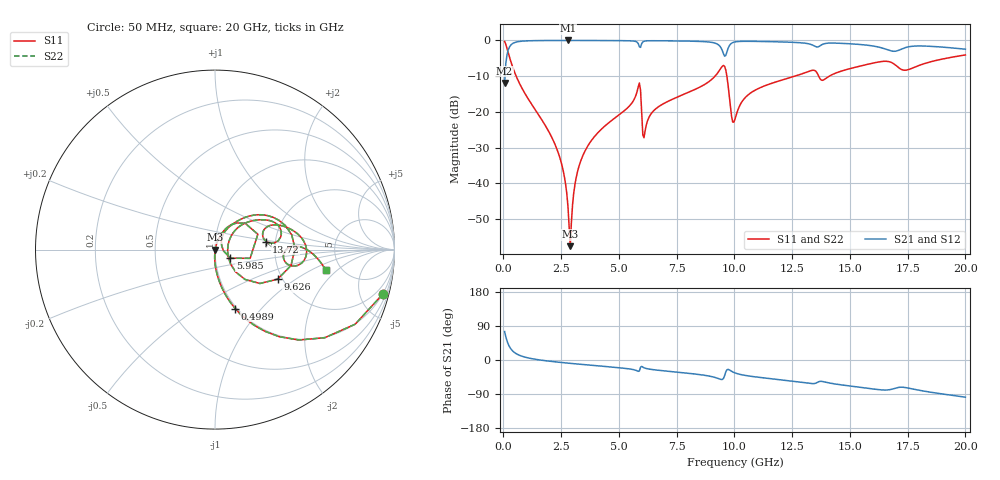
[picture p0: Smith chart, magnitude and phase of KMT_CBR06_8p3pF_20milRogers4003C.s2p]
! Data measured by Modelithics Inc. support@modelithics.com 813-866-6335
! KEMET CBR0603 8.3pF, Pad Width= 0.851mm, Pad Length= 0.64mm, Pad Gap= 0.62mm, 20mil Rogers 4003C substrate Data, January 2022
# hz S ma R 50
! 2 Port Network Data from SP1.SP block
! freq  magS11  angS11  magS21  angS21  magS12  angS12  magS22  angS22
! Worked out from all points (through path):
!   401 points, 50 MHz to 20 GHz, reference 50 ohm
!   highest |S21| = -0.01 dB at 2.793 GHz (marker M1); lowest = -11.9 dB at 50 MHz (marker M2)
!   group delay of S21, straight-line fit = 14.5 ps
!   lowest |S11| = -57.6 dB at 2.893 GHz (marker M3), VSWR 1.00, Z = 50.1 + j0.00236 ohm
!   |S11| at or under -10 dB: 550.4 MHz to 9.161 GHz (8.611 GHz wide, 177 % of centre); 9.674 GHz to 12.62 GHz (2.943 GHz wide, 26.4 % of centre); 13.65 GHz to 14.11 GHz (459.8 MHz wide, 3.31 % of centre)
!   |S22| runs from -57.6 to -0.3 dB; largest |S21 - S12| = 0
!   S11 on the Smith chart (normalised r, x): 50 MHz: 0.98, -7.53; 498.9 MHz: 0.98, -0.73; 5.985 GHz: 1.18, -0.11; 9.626 GHz: 1.89, -0.73; 13.72 GHz: 1.78, +0.17; 20 GHz: 3.79, -1.41
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5e7  0.967 -14.9  0.2542 75.1  0.2542 75.1  0.967 -14.9
2.495e8  0.6032 -53.6  0.7966 36.3  0.7966 36.3  0.6032 -53.6
4.98875e8  0.3471 -71.1  0.9369 18.8  0.9369 18.8  0.3471 -71.1
2.294375e9  0.03131 -93.1  0.9983 -5.2  0.9983 -5.2  0.03131 -93.1
2.593625e9  0.01468 -92.2  0.9986 -7.1  0.9986 -7.1  0.01468 -92.2
2.793125e9  0.004741 -82.6  0.9986 -8.3  0.9986 -8.3  0.004741 -82.6
2.892875e9  0.00132 1.0  0.9986 -8.8  0.9986 -8.8  0.00132 1.0
3.14225e9  0.01173 73.1  0.9985 -10.3  0.9985 -10.3  0.01173 73.1
3.391625e9  0.02252 74.8  0.9982 -11.6  0.9982 -11.6  0.02252 74.8
5.8355e9  0.2234 40.8  0.9036 -29.9  0.9036 -29.9  0.2234 40.8
5.985125e9  0.09822 -29.3  0.9036 -17.0  0.9036 -17.0  0.09822 -29.3
6.13475e9  0.05458 49.4  0.9807 -21.6  0.9807 -21.6  0.05458 49.4
6.73325e9  0.1192 60.9  0.9889 -27.3  0.9889 -27.3  0.1192 60.9
9.227e9  0.3348 35.1  0.8989 -47.3  0.8989 -47.3  0.3348 35.1
9.626e9  0.3858 -25.3  0.6152 -31.5  0.6152 -31.5  0.3858 -25.3
9.875375e9  0.08719 -30.8  0.9125 -29.7  0.9125 -29.7  0.08719 -30.8
1.0025e10  0.0794 21.7  0.9528 -34.0  0.9528 -34.0  0.0794 21.7
1.0823e10  0.1951 43.2  0.9704 -43.9  0.9704 -43.9  0.1951 43.2
1.336662e10  0.3813 18.7  0.8657 -62.2  0.8657 -62.2  0.3813 18.7
1.371575e10  0.2881 9.0  0.8441 -56.3  0.8441 -56.3  0.2881 9.0
1.670825e10  0.5029 -6.1  0.725 -78.5  0.725 -78.5  0.5029 -6.1
2e10  0.6264 -10.4  0.7533 -98.1  0.7533 -98.1  0.6264 -10.4
